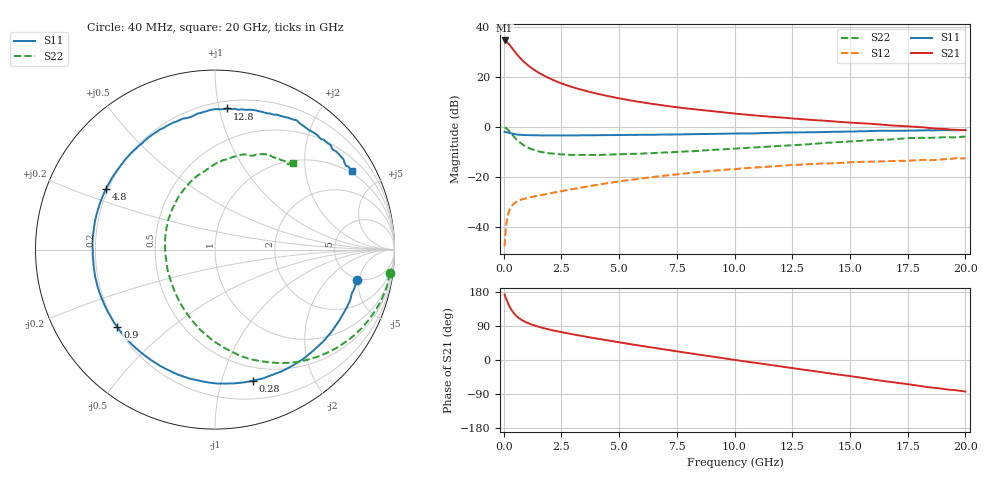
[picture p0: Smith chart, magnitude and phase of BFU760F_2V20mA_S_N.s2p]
! Filename:  P:\Prog\Test\Noise\ATS_data\Testdata_Net\BFU760\BFU760F_2W_C1_2V20mA_D.s2p
! Date/Time: Mon 06/Feb/2012 15:05:38
! BFU760_2W_C1_2V20mA
! bias mode 1: Vout= 2.0003 V, Iout=19.9650 mA, Vin= 0.7874 V, Iin= 0.0625 mA
! Date/time Fri Mar 18 14:39:14 2011
! Device data file deembeded for feedlines and parallel
! Original file: \BFU760\BFU760_2W_C1_2V20mA_R.s2p
! Feed-files: PR003V01_101208_Feed1.s2p, PR003V01_101208_Feed2.s2p
! Parallel-file: PR003V01_101208_Par.s2p
# MHz S MA R 50
!  Freq-MHz  S11-mag  S11-arg  S21-mag  S21-arg  S12-mag  S12-arg  S22-mag  S22-arg
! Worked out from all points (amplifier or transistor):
!   167 points, 40 MHz to 20 GHz, reference 50 ohm
!   highest |S21| = 34.8 dB at 40 MHz (marker M1)
!   |S21| within 3 dB of that: start of sweep to 357.9 MHz
!   unconditionally stable (mu >= 1): 4.326 GHz to 13.81 GHz
!   at 550 MHz: K = 0.24, MSG = 29.7 dB, |S12| = -29.9 dB
!   at 4.2 GHz: K = 0.99, MSG = 18.0 dB, |S12| = -22.9 dB
!   at 20 GHz: K = 0.89, MSG = 5.7 dB, |S12| = -12.5 dB
!   lowest NFmin = 0.51 dB at 400 MHz
!   S11 on the Smith chart (normalised r, x): 40 MHz: 4.82, -4.64; 280 MHz: 0.36, -1.26; 900 MHz: 0.20, -0.34; 4.8 GHz: 0.19, +0.25; 12.8 GHz: 0.25, +1.06; 20 GHz: 0.93, +3.52
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40  0.8073 -12.0  54.92 173.1  0.004115 82.1  0.9841 -7.8
50  0.8063 -15.6  54.74 170.8  0.005178 86.2  0.9803 -10.0
90  0.7986 -26.6  53.52 164.4  0.00909 77.0  0.9646 -18.1
160  0.7853 -45.7  49.99 153.6  0.01527 68.3  0.9111 -31.6
220  0.7743 -60.7  46.84 145.4  0.01964 61.9  0.8532 -41.9
280  0.7607 -73.9  43.28 138.2  0.02319 56.5  0.794 -51.1
340  0.7488 -85.4  39.82 132.1  0.02594 51.9  0.7342 -59.4
420  0.7336 -98.6  35.66 125.1  0.02882 47.1  0.6645 -68.8
550  0.717 -114.9  29.93 116.3  0.03191 41.9  0.5697 -81.6
700  0.7045 -128.4  24.85 109.0  0.03448 38.2  0.4939 -93.3
900  0.6949 -141.5  20.08 101.7  0.03684 35.7  0.4244 -105.8
1300  0.687 -157.9  14.36 91.8  0.04067 34.3  0.3499 -124.6
1850  0.6828 -171.7  10.22 82.2  0.04571 35.0  0.3057 -142.6
2500  0.6834 177.4  7.57 73.6  0.05213 36.4  0.2867 -157.9
3400  0.6871 165.9  5.593 63.3  0.06223 36.7  0.2778 -173.0
4800  0.6954 150.9  3.955 48.6  0.07929 34.6  0.2838 168.6
6800  0.7098 132.8  2.778 29.4  0.1046 27.5  0.3076 147.7
10200  0.7492 104.9  1.84 -1.5  0.1474 9.9  0.3774 117.6
12800  0.7893 85.0  1.465 -23.8  0.1777 -5.7  0.4424 97.0
13400  0.7902 80.5  1.395 -28.9  0.1837 -10.2  0.4627 92.6
16800  0.8466 54.6  1.085 -58.1  0.209 -31.8  0.5687 67.3
20000  0.8776 29.9  0.8729 -83.3  0.2375 -53.4  0.6473 48.0
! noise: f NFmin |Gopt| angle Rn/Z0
400  0.5051  0.09678  159.9  0.0453
650  0.5086  0.1159  155.6  0.0471
1050  0.5162  0.1465  153.5  0.0492
1450  0.5262  0.1761  154.4  0.0505
1900  0.5404  0.2082  157.6  0.051
2350  0.5576  0.2399  162  0.0507
3000  0.5879  0.287  169.7  0.049
3800  0.6339  0.3521  180.2  0.0455
4600  0.6896  0.4303  190.8  0.0412
6000  0.8102  0.6098  207.3  0.0338
